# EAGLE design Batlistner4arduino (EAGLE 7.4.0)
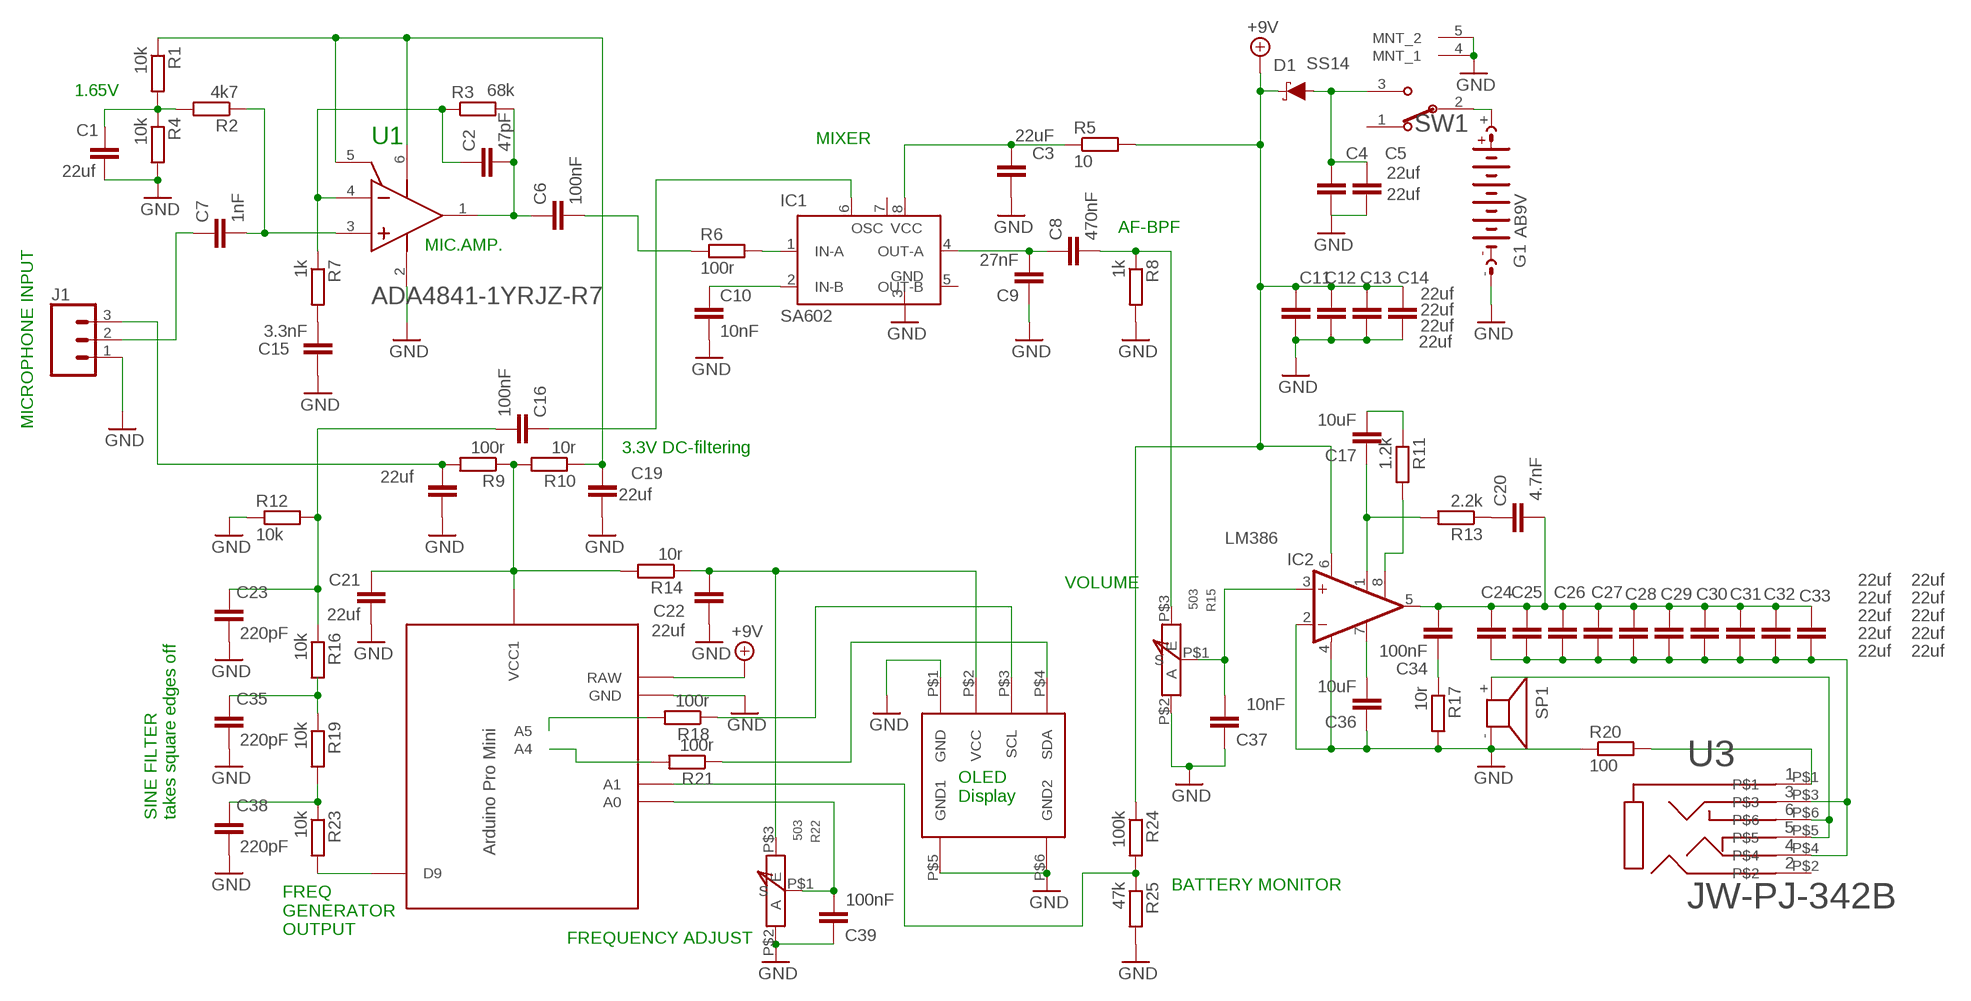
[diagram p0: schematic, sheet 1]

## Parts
C1  22uf  C-EUC0805  [C0805]
C2  47pF  C-EUC0805  [C0805]
C3  22uF  C-EUC0805  [C0805]
C4  22uf  C-EUC0805  [C0805]
C5  22uf  C-EUC0805  [C0805]
C6  100nF  C-EUC0805  [C0805]
C7  1nF  C-EUC0805  [C0805]
C8  470nF  C-EUC0805  [C0805]
C9  27nF  C-EUC0805  [C0805]
C10  10nF  C-EUC0805  [C0805]
C11  22uf  C-EUC0805  [C0805]
C12  22uf  C-EUC0805  [C0805]
C13  22uf  C-EUC0805  [C0805]
C14  22uf  C-EUC0805  [C0805]
C15  3.3nF  C-EUC0805  [C0805]
C16  100nF  C-EUC0805  [C0805]
C17  10uF  C-EUC0805  [C0805]
C18  22uf  C-EUC0805  [C0805]
C19  22uf  C-EUC0805  [C0805]
C20  4.7nF  C-EUC0805  [C0805]
C21  22uf  C-EUC0805  [C0805]
C22  22uf  C-EUC0805  [C0805]
C23  220pF  C-EUC0805  [C0805]
C24  22uf  C-EUC0805  [C0805]
C25  22uf  C-EUC0805  [C0805]
C26  22uf  C-EUC0805  [C0805]
C27  22uf  C-EUC0805  [C0805]
C28  22uf  C-EUC0805  [C0805]
C29  22uf  C-EUC0805  [C0805]
C30  22uf  C-EUC0805  [C0805]
C31  22uf  C-EUC0805  [C0805]
C32  22uf  C-EUC0805  [C0805]
C33  22uf  C-EUC0805  [C0805]
C34  100nF  C-EUC0805  [C0805]
C35  220pF  C-EUC0805  [C0805]
C36  10uF  C-EUC0805  [C0805]
C37  10nF  C-EUC0805  [C0805]
C38  220pF  C-EUC0805  [C0805]
C39  100nF  C-EUC0805  [C0805]
D1  SS14  DIODE-SCHOTTKY-SS14  [SMA-DIODE]
G1  AB9V  [AB9V]
IC1  SA602  SA612AD  [SO08]
IC2  LM386  LM386M-1  [SO08]
J1  CONN_03  [1X03]
R1  10k  R-EU_M0805  [M0805]
R2  4k7  R-EU_M0805  [M0805]
R3  68k  R-EU_M0805  [M0805]
R4  10k  R-EU_M0805  [M0805]
R5  10  R-EU_M0805  [M0805]
R6  100r  R-EU_M0805  [M0805]
R7  1k  R-EU_M0805  [M0805]
R8  1k  R-EU_M0805  [M0805]
R9  100r  R-EU_M0805  [M0805]
R10  10r  R-EU_M0805  [M0805]
R11  1.2k  R-EU_M0805  [M0805]
R12  10k  R-EU_M0805  [M0805]
R13  2.2k  R-EU_M0805  [M0805]
R14  10r  R-EU_M0805  [M0805]
R15  503  RK10J11SINGE  [RK10J11]
R16  10k  R-EU_M0805  [M0805]
R17  10r  R-EU_R1210  [R1210]
R18  100r  R-EU_M0805  [M0805]
R19  10k  R-EU_M0805  [M0805]
R20  100  R-EU_R0805  [R0805]
R21  100r  R-EU_M0805  [M0805]
R22  503  RK10J11SINGE  [RK10J11]
R23  10k  R-EU_M0805  [M0805]
R24  100k  R-EU_M0805  [M0805]
R25  47k  R-EU_M0805  [M0805]
SP1  PADSONLY  [PADSONLY]
SW1  EG1206A  E-SWITCH_EG1206AE-SWITCH_EG1206A_0_0  [E-SWITCH_EG1206A_0]
U1  ADA4841  ANALOG_DEVICES_ADA4841-1YRJZ-R7ANALOG_DEVICES_ADA4841-1YRJZ-R7_0_1  [ANALOG_DEVICES_ADA4841-1YRJZ-R7_1]
U2  PRO-MINI-2  [PRO-MINI-2]
U3  JW-PJ-342B  [JW-PJ-342B]
U4  OLED  [SIP]

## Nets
+9V: C11.1 C12.1 C13.1 C14.1 D1.C IC2.6(VS) R5.2 R24.1 U2.RAW
GND: C1.2 C3.1 C4.2 C5.2 C9.1 C10.2 C11.2 C12.2 C13.2 C14.2 C15.1 C18.2 C19.2 C21.2 C22.2 C23.2 C35.2 C36.1 C37.1 C38.2 C39.1 G1.- IC1.3(GND) IC2.2(-IN) IC2.4(GND) J1.1 R4.2 R8.2 R12.1 R15.P$2(A) R17.2 R20.1 R22.P$2(A) R25.2 SP1.- SW1.4(MNT_1) SW1.5(MNT_2) U1.2(-VS) U2.GND U4.P$1(GND) U4.P$5(GND1) U4.P$6(GND2)
N$1: C24.2 C25.2 C26.2 C27.2 C28.2 C29.2 C30.2 C31.2 C32.2 C33.2 U3.P$3 U3.P$4
N$2: C34.1 R17.1
N$3: C1.1 R1.2 R2.2 R4.1
N$4: C36.2 IC2.7(BYPASS)
N$5: C8.1 C9.2 IC1.4(OUT-A)
N$6: C21.1 R9.1 R10.2 R14.2 U2.VCC1
N$7: C18.1 J1.3 R9.2
N$8: C7.2 R2.1 U1.3(+IN)
N$9: C4.1 C5.1 D1.A SW1.3
N$10: C19.1 R1.1 R10.1 U1.5(!POWER_DOWN!) U1.6(+VS)
N$11: C2.1 R3.1 R7.1 U1.4(-IN)
N$12: C2.2 C6.1 R3.2 U1.1(VOUT)
N$13: C7.1 J1.2
N$14: C6.2 R6.1
N$15: C15.2 R7.2
N$16: C22.1 R14.1 R22.P$3(E) U4.P$2(VCC)
N$17: C39.2 R22.P$1(S) U2.A0
N$18: IC1.1(IN-A) R6.2
N$19: C10.1 IC1.2(IN-B)
N$20: C8.2 R8.1 R15.P$3(E)
N$21: R21.1 U4.P$4(SDA)
N$22: C37.2 IC2.3(+IN) R15.P$1(S)
N$23: R18.1 U4.P$3(SCL)
N$24: R24.2 R25.1 U2.A1
N$25: C16.2 C23.1 R12.2 R16.1
N$26: R23.2 U2.D9
N$27: C20.1 C24.1 C25.1 C26.1 C27.1 C28.1 C29.1 C30.1 C31.1 C32.1 C33.1 C34.2 IC2.5(OUT)
N$28: C38.1 R19.2 R23.1
N$29: C35.1 R16.2 R19.1
N$30: C16.1 IC1.6(OSC)
N$31: R21.2 U2.A4
N$32: R18.2 U2.A5
N$50: C20.2 R13.1
N$56: C17.1 IC2.1(GAIN) R13.2
N$59: C3.2 IC1.8(VCC) R5.1
N$61: C17.2 R11.1
N$62: IC2.8(GAIN) R11.2
N$64: R20.2 U3.P$1
N$65: SP1.+ U3.P$5 U3.P$6
N$67: G1.+ SW1.2(COM)
Unconnected: IC1.5(OUT-B) IC1.7(OSC') SW1.1 U3.P$2

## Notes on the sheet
- 1.65V
- MIXER
- AF-BPF
- MIC.AMP.
- MICROPHONE INPUT
- 3.3V DC-filtering
- VOLUME
- OLED
  Display
- SINE FILTER
  takes square edges off
- BATTERY MONITOR
- FREQ
  GENERATOR
  OUTPUT
- FREQUENCY ADJUST

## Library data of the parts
C1-C39 = rcl:C-EU: CAPACITOR, European symbol
D1 = SparkFun-DiscreteSemi:DIODE-SCHOTTKY: Schottky diode; PROD_ID: DIO-08053; VALUE: 1A/40V/500mV
G1 = battery:AB9V: 9-V BATTERY CLIP
IC1 = linear:SA612A: Double-balanced mixer and oscillator NE612/SA612 Source: www-eu2.semiconductors.philips.com/acrobat/datasheets/SA612A.pdf
IC2 = linear:LM386?-*: Low Voltage Audio Power Amplifier Source: http://cache.national.com/ds/LM/LM386.pdf
J1 = SparkFun-Connectors:CONN_03: Multi connection point. Often used as Generic Header-pin footprint for 0.1 inch spaced/style header connections On any of the 0.1 inch spaced packages, you can populate with these: Break Away Headers - Straight (PRT-00116) Break Away Male Headers - Right Angle (PRT-00553) Female Headers (PRT-00115)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; PROD_ID: XXX-00000; VALUE: 455-1750-1-ND
R1-R14 R16-R21 R23-R25 = rcl:R-EU_: RESISTOR, European symbol
R15 R22 = pe1pwf:RK10J11: Thumb wheel potentiometer
SP1 = buzzer1:PADSONLY: Speakerpads
SW1 = E-Switch - EG1206A:E-SWITCH_EG1206A: Slide Switch SPDT 200mA 30V; CENTROID_NOT_SPECIFIED: No; DATASHEET: http://spec_sheets.e-switch.com/specs/P040021.pdf; DIGIKEY_DESCRIPTION: SWITCH Slide Switch SPDT Through Hole, Right Angle; DIGIKEY_PART_NUMBER: EG1917-ND; LEAD_FREE: yes; MF: E-Switch; MOUSER_PART_NUMBER: 612-EG1206A; MPN: EG1206A; PACKAGE: SIP; PREFIX: SW; ROHS: yes; TEMPERATURE_RANGE_HIGH: +70°C; TEMPERATURE_RANGE_LOW: -20°C
U1 = Analog Devices - ADA4841-1YRJZ-R7:ANALOG_DEVICES_ADA4841-1YRJZ-R7: ADI-ADA48X1-1-RJ-6; AMPLIFIERS_PER_PACKAGE: 1; CIIVA_IDS: 1319929; CODE__JEDEC: MO-178-AB; COMPONENT_LINK_1_DESCRIPTION: Manufacturer URL; COMPONENT_LINK_1_URL: http://www.analog.com/en/index.html; COMPONENT_LINK_3_DESCRIPTION: Package Specification; COMPONENT_LINK_3_URL: http://www.analog.com/static/imported-files/packages/PKG_PDF/SOT-23(RJ)/RJ_6.pdf; COMPONENT_LINK_4_DESCRIPTION: Reference Circuit; COMPONENT_LINK_4_URL: http://www.analog.com/en/all-operational-amplifiers-op-amps/operational-amplifiers-op-amps/ada4841-1/products/product.html#product-recommendations; DATASHEET: http://www.analog.com/static/imported-files/data_sheets/ADA4841-1_4841-2.pdf; DATASHEET_VERSION: Rev. E; FOOTPRINT_VARIANT_NAME_0: Level C; FOOTPRINT_VARIANT_NAME_1: Level B; FOOTPRINT_VARIANT_NAME_2: Level A; IMPORTED: yes; IMPORTED_FROM: vault; IMPORT_TS: 1521849189; INPUT_BIAS_CURRENT: 3uA; INPUT_OFFSET_VOLTAGE: 40uV; IQ_AMP: 1.5mA; MF: Analog Devices; MOUNTING_TECHNOLOGY: Surface Mount; MPN: ADA4841-1YRJZ-R7; PACKAGE: RJ-6; PACKAGE_DESCRIPTION: 6-Pin Small Outline Transistor Package, Body 2.9 x 1.6 mm, Pitch 0.95 mm; PACKAGE_VERSION: 121608-A; PREFIX: U; RELEASE_DATE: 1386929931; SLEW_RATE: 13V/us; SMALL_SIGNAL_BANDWIDTH: 80MHz; VAULT_GUID: F126E6A0-1EF3-4483-8FCE-B4A852E3AD50; VAULT_REVISION: 933F59B0-58C5-4864-91C7-6571D66461B8; V_SPAN_MAX: 12V; V_SPAN_MIN: 2.7V
U2 = Arduino-clone:PRO-MINI-2: Arduino Pro Mini Layout 2 Sparkfun.com
U3 = jack:JW-PJ-342B
U4 = OLED042:OLED: I2C 0.91"128x32 OLED

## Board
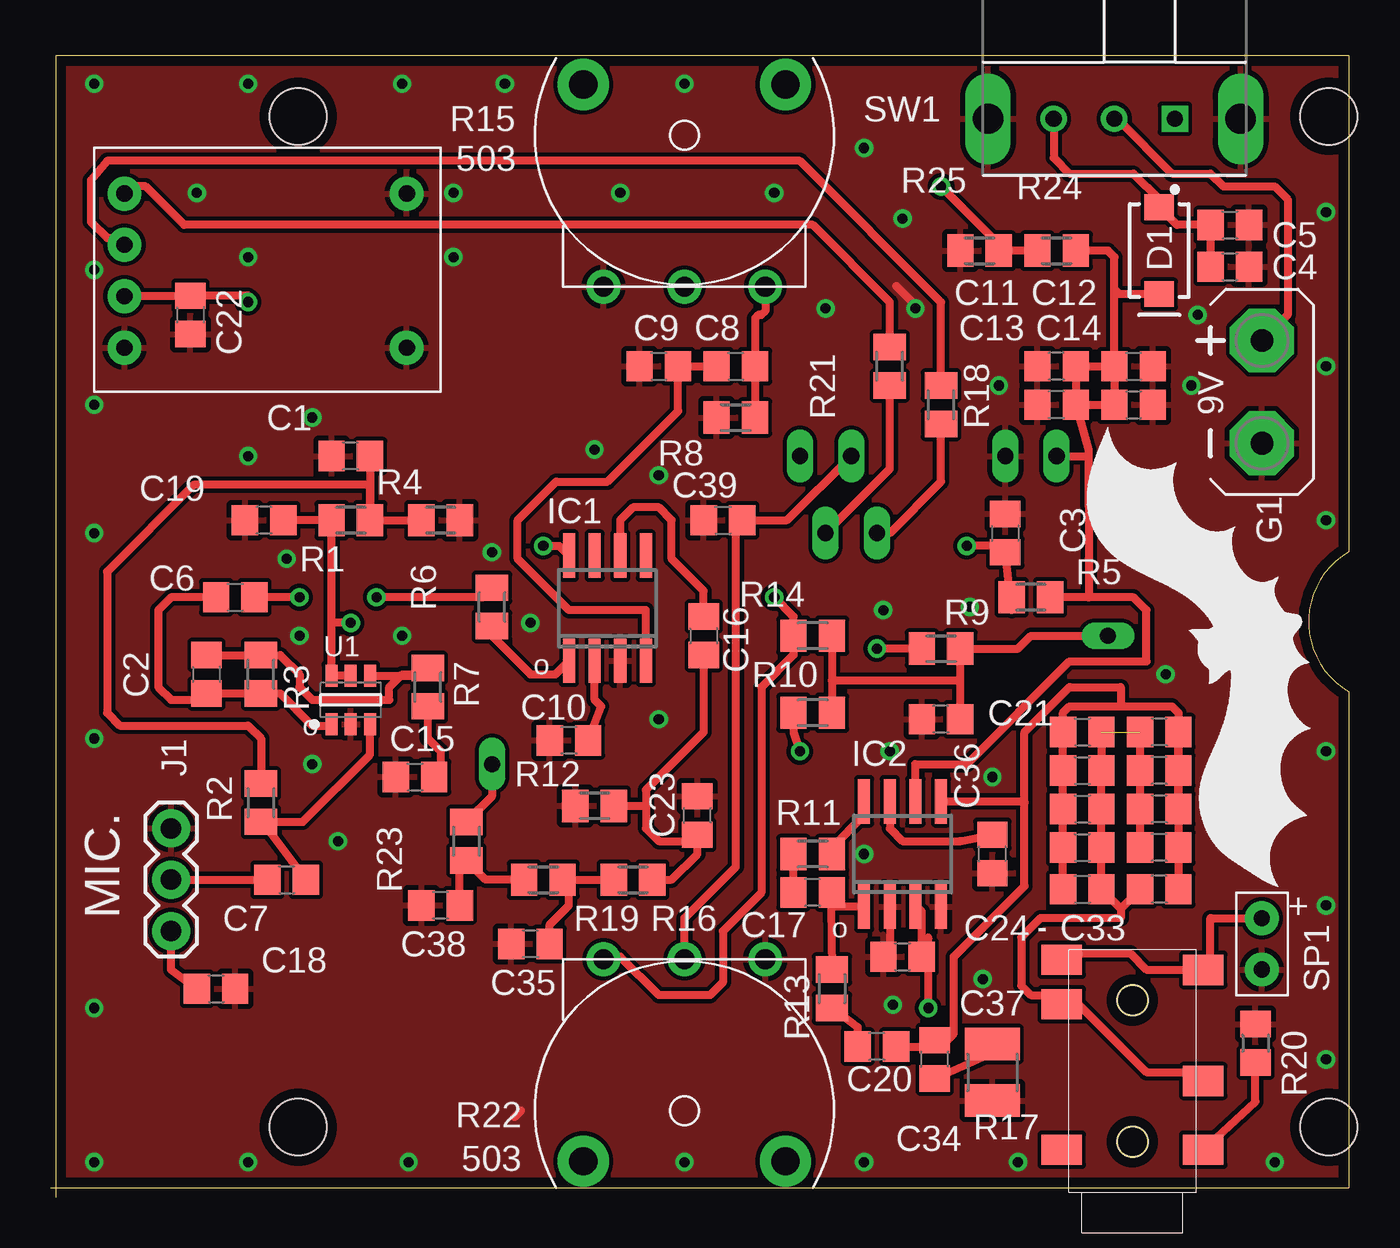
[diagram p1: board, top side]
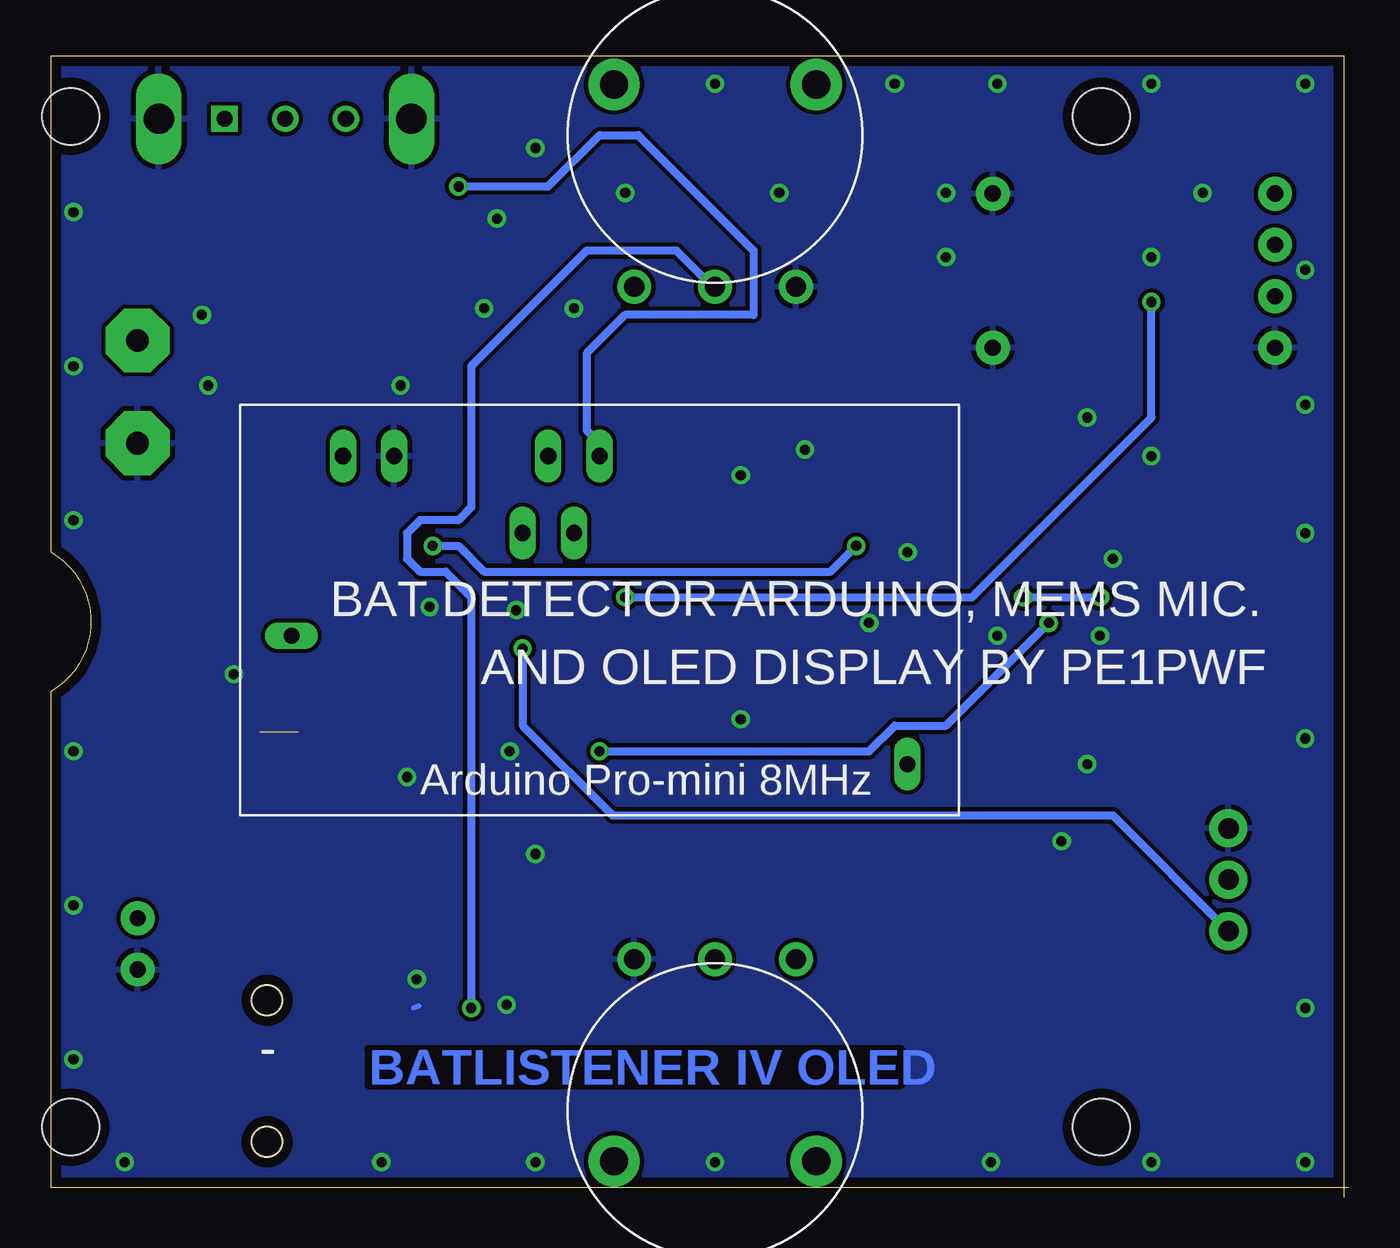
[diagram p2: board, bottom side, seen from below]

Size 64.25 x 56.47 mm. Coordinates in mm from the lower left corner, seen from the top.
Outline: 0.25,0 0.25,56.47 64.25,56.47 64.25,31.93 arc120 64.25,25 64.25,0.47 0,0.47
Copper layers (1*16): Top 0.035mm / dielectric 1.5mm / Bottom 0.035mm
Design rules "default *": minimum track width 10mil, minimum drill 19mil, track to track 8mil, track to pad 8mil, pad to pad 8mil, via to via 8mil, smd to smd 8mil, copper to edge 20mil, drill to drill 8mil, minimum pad ring 10mil, minimum via ring 8mil, stop-mask expansion 4mil, vias tented up to drill 20mil, thermal gap 10mil
Holes 2.8 mm at 63.25,3.46 63.25,53.47 12.25,53.47 12.25,3.46

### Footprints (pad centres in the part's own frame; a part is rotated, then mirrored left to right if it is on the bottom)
C0805 = smd 1.3 x 1.5: 1 -0.95,0; 2 0.95,0
SMA-DIODE = smd 1.27 x 1.47: A -2.15,0; C 2.15,0
AB9V = drill 1.118 pad 3.15 octagon: + 0,2.54; - 0,-2.54
SO08 = smd 0.6 x 2.2: 1 -1.905,-2.6; 2 -0.635,-2.6; 3 0.635,-2.6; 4 1.905,-2.6; 5 1.905,2.6; 6 0.635,2.6; 7 -0.635,2.6; 8 -1.905,2.6
1X03 = drill 1.016 pad 1.88: 1 0,0; 2 2.54,0; 3 5.08,0
M0805 = smd 1.3 x 1.6: 1 -0.95,0; 2 0.95,0
RK10J11 = drill 1 pad 1.676: P$1 0,-7.5; P$2 -4,-7.5; P$3 4,-7.5 | drill 1.4 pad 2.54: P$4 5,2.5; P$5 -5,2.5
R1210 = smd 1.6 x 2.7: 1 -1.4,0; 2 1.4,0
R0805 = smd 1.3 x 1.5: 1 -0.95,0; 2 0.95,0
PADSONLY = drill 0.8 pad 1.676: + 0,0; - 0,-2.54
E-SWITCH_EG1206A_0 = drill 0.8 pad 1.3 square: 1 -3,3 | drill 0.8 pad 1.3: 2 0,3; 3 3,3 | drill 1.5 pad 1.778 long: 4 -6.25,3; 5 6.25,3
ANALOG_DEVICES_ADA4841-1YRJZ-R7_1 = smd 1.1 x 0.6: 1 -1.2,0.95; 2 -1.2,0; 3 -1.2,-0.95; 4 1.2,-0.95; 5 1.2,0; 6 1.2,0.95
PRO-MINI-2 = drill 0.8 long: A0 6.35,2.54; A1 6.35,0; A4 2.54,1.27; A5 2.54,3.81; D9 -8.89,-15.24; GND 6.35,10.16; RAW 6.35,12.7; VCC1 -2.54,15.24
JW-PJ-342B = smd 1.5 x 2: P$1 4.1,1; P$2 4.1,8; P$3 7.5,1; P$4 11.3,8; P$5 13.5,8; P$6 13,1 | hole 1.5: 4.5,4.5; 11.5,4.5
SIP = drill 0.8 pad 1.676: P$1 -17.55,-4.16; P$2 -17.55,-1.62; P$3 -17.55,0.92; P$4 -17.55,3.46; P$5 -3.58,-4.16; P$6 -3.58,3.46

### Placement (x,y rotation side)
C1  14.86,36.66 180 top
C2  7.72,25.86 270 top
C3  47.24,32.85 270 top
C4  58.36,46.03 0 top
C5  58.36,48.09 0 top
C6  9.14,29.68 0 top
C7  11.68,15.71 0 top
C8  33.91,41.11 0 top
C9  30.1,41.11 0 top
C10  25.65,22.59 180 top
C11  53.59,41.11 0 top
C12  53.59,39.2 0 top
C13  49.78,41.11 180 top
C14  49.78,39.2 180 top
C15  18.03,20.79 0 top
C16  32.32,27.77 270 top
C17  37.72,15.07 180 top
C18  8.19,10.31 0 top
C19  10.57,33.49 180 top
C20  40.89,7.45 180 top
C21  44.07,23.64 180 top
C22  6.92,43.65 270 top
C23  32,18.88 90 top
C24  51.05,15.23 0 top
C25  54.86,15.23 180 top
C26  54.86,17.29 180 top
C27  54.86,19.2 180 top
C28  54.86,21.1 180 top
C29  54.86,23.01 180 top
C30  51.05,23.01 0 top
C31  51.05,21.1 0 top
C32  51.05,19.2 0 top
C33  51.05,17.29 0 top
C34  43.75,6.81 90 top
C35  23.75,12.53 180 top
C36  46.61,16.98 90 top
C37  42.16,11.89 0 top
C38  19.3,14.44 180 top
C39  33.27,33.49 0 top
D1  54.86,46.82 270 top
G1  59.94,39.84 0 top
IC1  27.56,29.14 0 top
IC2  42.16,16.98 0 top
J1  5.97,18.25 270 top
R1  14.86,33.49 0 top
R2  10.41,19.52 90 top
R3  10.41,25.86 270 top
R4  19.3,33.49 0 top
R5  48.51,29.68 0 top
R6  21.84,29.2 270 top
R7  18.67,25.23 270 top
R8  33.91,38.57 180 top
R9  44.07,27.14 180 top
R10  37.72,23.96 0 top
R11  37.72,16.98 0 top
R12  26.92,19.36 0 top
R13  38.67,10.31 90 top
R14  37.72,27.77 0 top
R15  31.37,52.54 0 top
R16  28.83,15.71 180 top
R17  46.61,6.18 270 top
R18  44.07,39.2 270 top
R19  24.38,15.71 180 top
R20  59.63,7.61 270 top
R21  41.53,41.11 270 top
R22  31.37,4.28 180 top
R23  20.57,17.61 90 top
R24  49.78,46.82 180 top
R25  45.97,46.82 180 top
SP1  59.94,13.8 0 top
SW1  52.64,56.35 180 top
U1  14.86,24.59 90 top
U2  37.08,30.31 90 bottom
U3  58.04,-1.76 90 top
U4  21.21,46.19 0 top

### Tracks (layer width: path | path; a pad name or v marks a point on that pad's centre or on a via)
+9V
  Top 0.406: C11.1 C12.1 | C14.1 51.37,36.98 51.37,36.66 | 51.37,36.66 51.37,31.58 51.37,29.68 R5.2 53.59,29.68 54.23,29.04 54.23,26.5 54.07,26.5 50.42,26.5 45.34,21.42 42.8,21.42 IC2.6 | C14.1 C13.1 C11.1 | 50.42,39.2 C14.1 | C14.1 52.96,39.2 | C11.1 52.64,44.92 | 52.64,44.92 52.64,46.5 52.32,46.82 R24.1 | D1.C 52.89,44.67 52.64,44.92 | U2.RAW 51.37,36.66 | 51.37,36.66
GND  (via drill 0.5)
  Top 0.406: IC2.2 41.53,12.21 C37.1 | 23.27,4.28 22.96,3.96 | 42.8,43.8 42.8,44.12 41.85,45.07
  Bottom 0.254: 46,9.46 46.29,9.36
  other vias: 46.93,40.15 2.16,55.08 9.78,55.08 17.4,55.08 22.48,55.08 2.16,39.2 9.78,1.74 40.26,1.74 47.88,1.74 60.58,1.74 63.12,6.81 63.12,14.44 63.12,22.05 63.12,33.49 63.12,41.11 63.12,48.73 31.37,55.08 40.26,16.98 46.61,20.79 46.13,10.78 55.18,25.86 42.16,48.41 38.35,43.96 2.16,45.87 56.77,43.65 42.8,43.96 7.24,49.68 28.19,49.68 11.68,31.58 12.95,21.42 19.94,49.68 19.94,46.5 9.78,46.5 12.32,27.77 17.4,27.77 23.75,28.41 14.22,17.61 2.16,1.74 2.16,32.85 2.16,22.69 2.16,9.36 21.84,31.9 26.92,36.98 30.1,35.71 30.1,23.64 56.45,40.15 40.26,51.9 17.72,1.74 31.37,1.74 35.81,49.68 41.21,29.04 41.53,22.05 41.69,9.51 45.5,29.2 9.78,36.66 12.95,38.57
  pour Top: 6.6,-0.17 0.25,0.47 0.25,56.35 64.39,56.35 64.39,32.22 62.48,28.41 65.02,24.59 64.39,0.47
  pour Bottom: 64.39,0.47 0.25,-0.17 0.25,56.35 65.02,56.35 65.02,32.22 62.48,28.41 65.02,24.59
N$1  (1 unrouted)
  Top 0.406: C29.2 C28.2 C27.2 C26.2 | C30.2 C31.2 C32.2 C33.2 C24.2 52.96,14.28 | 52.96,14.28 C25.2 | 52.96,14.28 52.96,13.8 48.99,13.8 48.04,12.85 48.04,10.47 48.51,9.99 49.91,9.99 U3.P$4 50.55,9.86 54.23,6.18 56.92,6.18 U3.P$3
N$2
  Top 0.406: C34.1 46.6,7.13 R17.1
N$3
  Top 0.406: C1.1 R1.2 | R1.2 R4.1 | R1.2 15.81,35.23 7.08,35.23 2.79,30.95 2.79,23.96 3.43,23.32 9.78,23.32 10.41,22.69 R2.2 10.09,20.79
N$4
  Top 0.406: IC2.7 41.53,18.25 42.16,17.61 45.02,17.61 C36.2
N$5
  Top 0.406: C8.1 C9.2 31.05,38.88 27.56,35.39 25.02,35.39 23.11,33.49 23.11,31.58 25.65,29.04 29.46,29.04 IC1.4
N$6
  Top 0.406: U2.VCC1 48.51,27.77 47.88,27.14 R9.1 C21.1 45.02,25.39 45.02,25.55 38.67,25.55 | R14.2 38.67,25.55 | 38.67,25.55 R10.2
N$7  (via drill 0.5)
  Top 0.406: R9.2 v40.89,27.14 | C18.1 5.97,11.26 J1.3
  Bottom 0.406: v40.89,27.14 40.89,23.32 36.45,18.88 11.68,18.88 J1.3
N$8
  Top 0.406: C7.2 10.73,18.25 R2.1 12.48,18.57 15.81,21.9 U1.3
N$9
  Top 0.406: SW1.3 49.64,51.41 50.42,50.63 53.59,50.63 54.86,49.36 D1.A 55.74,48.09 C5.1 C4.1
N$10  (via drill 0.5)
  Top 0.406: U1.5 U1.6 13.91,28.41 | 13.91,28.41 R1.1 C19.1 | R10.1 36.77,23.01 v37.08,22.05 | v14.86,28.41 13.91,28.41
  Bottom 0.406: v37.08,22.05 23.75,22.05 22.48,23.32 19.94,23.32 v14.86,28.41
N$11
  Top 0.406: C2.1 R3.1 11.37,26.82 12.32,25.86 12.32,25.23 12.95,24.59 16.76,24.59 16.76,25.23 17.4,25.86 18.35,25.86 R7.1 18.28,25.79 U1.4
N$12
  Top 0.406: C6.1 5.97,29.68 5.33,29.04 5.33,25.23 5.97,24.59 7.39,24.59 C2.2 R3.2 11.36,24.91 12.95,23.32 13.84,23.32 U1.1
N$13
  Top 0.406: J1.2 C7.1
N$14  (via drill 0.5)
  Top 0.406: R6.1 21.37,29.68 v16.13,29.68 | v12.32,29.68 C6.2
  Bottom 0.406: v16.13,29.68 v12.32,29.68
N$15
  Top 0.406: R7.2 18.67,22.69 19.3,22.05 19.3,21.11 C15.2
N$16  (via drill 0.5)
  Top 0.406: v35.81,29.68 36.77,28.72 R14.1 36.77,26.82 35.18,25.23 35.18,15.07 33.27,13.16 33.27,10.62 32.64,9.99 30.1,9.99 28.19,11.89 27.49,11.89 R22.P$3 | v9.78,44.28 9.78,44.6 C22.1 6.92,44.57 U4.P$2
  Bottom 0.406: v35.81,29.68 18.67,29.68 9.78,38.57 v9.78,44.28
N$17
  Top 0.406: R22.P$1 31.37,13.8 33.91,16.34 33.91,33.17 C39.2 36.45,33.49 U2.A0
N$18
  Top 0.406: R6.2 21.84,27.77 23.75,25.86 24.98,25.86 IC1.1
N$19
  Top 0.406: C10.1 27.24,24.27 26.92,24.59 IC1.2
N$20
  Top 0.406: R8.1 C8.2 34.86,43.49 35.02,43.65 35.18,43.65 35.37,43.84 R15.P$3
N$21
  Top 0.406: R21.1 41.53,44.28 37.72,48.09 6.6,48.09 4.7,50 4.01,50 U4.P$4
N$22  (via drill 0.5)
  Top 0.406: v43.43,9.36 43.43,12.85 C37.2 43.11,14.12 42.8,14.44 IC2.3
  Bottom 0.406: R15.P$1 31.49,45.04 33.27,46.82 37.72,46.82 43.43,41.11 43.43,34.12 44.07,33.49 45.97,33.49 46.61,32.85 46.61,31.58 45.97,30.95 44.7,30.95 43.43,29.68 v43.43,9.36
N$23
  Top 0.406: R18.1 44.07,44.28 37.08,51.27 2.79,51.27 2,50.31 2,48.25 2.79,47.46 3.31,47.46 U4.P$3
N$24  (via drill 0.5)
  Top 0.406: R24.2 R25.1 46.92,47.14 v44.07,50
  Bottom 0.406: v44.07,50 39.62,50 37.08,52.54 35.18,52.54 29.46,46.82 29.46,43.65 35.81,43.65 37.72,41.74 37.72,37.93 37.08,37.3 U2.A1
N$25
  Top 0.406: R16.1 30.73,15.71 32,16.98 C23.1 31.68,17.61 30.1,17.61 29.46,18.25 29.46,19.36 | C16.2 32.32,23.01 29.46,20.15 29.46,19.36 | R12.2 29.46,19.36
N$26
  Top 0.406: U2.D9 21.84,19.83 R23.2
N$27
  Top 0.406: C20.1 43.44,7.45 C34.2 44.38,7.76 44.7,8.09 44.7,11.89 45.34,12.53 48.2,15.39 48.2,19.52 | 48.2,19.52 48.2,23.01 50.42,25.23 52.96,25.23 52.96,24.28 | 52.96,24.28 55.5,24.28 55.82,23.96 55.82,19.52 C29.1 C28.1 C27.1 C26.1 C25.1 | C24.1 C33.1 C32.1 C31.1 C30.1 50.1,23.96 50.42,24.28 52.96,24.28 | IC2.5 48.14,19.57 48.2,19.52
N$28
  Top 0.406: C38.1 20.25,16.34 R23.1 21.53,15.71 R19.2
N$29
  Top 0.406: C35.1 24.7,13.48 25.65,14.44 25.65,15.38 R19.1 R16.2
N$30
  Top 0.406: C16.1 32.32,29.99 30.73,31.58 30.73,33.49 30.1,34.12 28.83,34.12 28.19,33.49 IC1.6
N$31
  Top 0.406: U2.A4 41.53,36.03 R21.2
N$32
  Top 0.406: U2.A5 41.53,32.85 44.07,35.39 R18.2
N$50
  Top 0.406: R13.1 39.94,8.41 C20.2
N$56
  Top 0.406: IC2.1 38.61,14.38 | 38.61,14.38 R13.2 | 38.61,14.38 38.61,15.02 C17.1
N$59  (via drill 0.5)
  Top 0.406: R5.1 47.56,29.04 C3.2 47.24,32.22 v45.34,32.22 | v24.38,32.22 25.17,32.22 IC1.8
  Bottom 0.406: v45.34,32.22 44.07,32.22 42.8,30.95 25.65,30.95 v24.38,32.22
N$61
  Top 0.406: C17.2 R11.1
N$62
  Top 0.406: R11.2 38.67,17.29 40.26,18.88 IC2.8
N$64
  Top 0.406: U3.P$1 59.63,4.72 R20.2
N$65
  Top 0.406: U3.P$5 50.27,11.74 50.58,12.05 53.43,12.06 54.23,11.26 56.74,11.26 U3.P$6 57.7,11.56 57.4,11.56 57.4,13.8 SP1.+
N$67
  Top 0.406: SW1.2 52.78,53.35 55.5,50.63 57.4,50.63 58.04,50 60.58,50 61.21,49.36 61.21,43.65 G1.+

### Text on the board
Bottom: BATLISTENER IV OLED
tPlace: -
tNames: o | o | MIC. | o
bNames: BAT DETECTOR ARDUINO, MEMS MIC. | AND OLED DISPLAY BY PE1PWF | Arduino Pro-mini 8MHz | -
